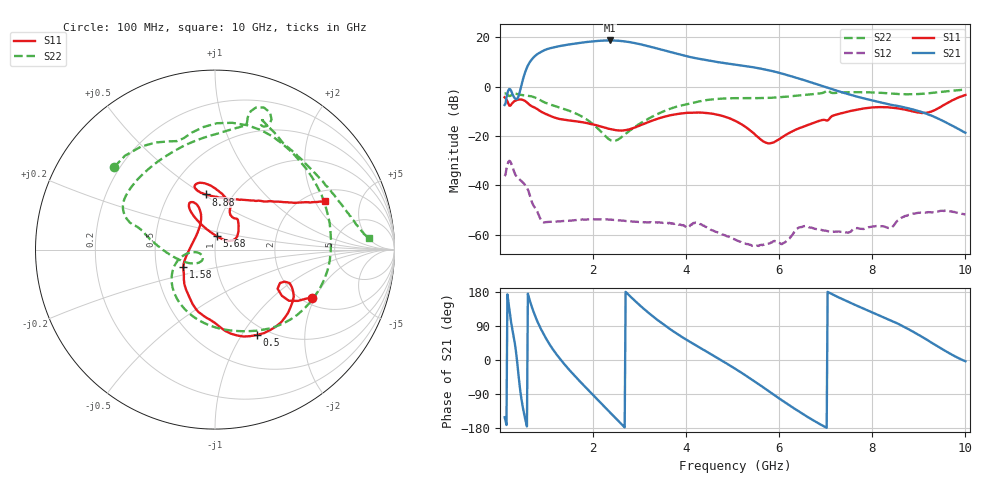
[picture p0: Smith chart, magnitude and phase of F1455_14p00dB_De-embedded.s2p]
! Integrated Device Technology
! Corporate Headquarters
! 6024 Silver Creek Valley Road
! San Jose, CA 95138  USA
! Phone:  1-408-284-8200
! Toll Free:  1-800-223-1366
! Webpage:  http://www.idt.com/
! Timing and RF Division
! 515 Groton Road, Suite 102
! Westford, MA 01886-6024
! Device:  F1455
! Description: 6-bit 0.5 dB Transmit Variable Gain Amplifier
! Frequency:  1400.0 -  2300.00 MHz
! Package:  6x6 mm Thin QFN Plastic Package: 28 pin
! State:  28
! Atten State:  14.0 dB
! Voltage:  +5.00 Volts
! Current:  217.654 mA
! Data:  The device was measured on a the F1455 evaluation board which has
!  individual transmission lines to the RF pins.  Data was collected
!  using a calibrated network analyzer.  The evaluation board was
!  de-embedded using a TRL calibration technique.
!  The reference plane is the edge of the package pin.
!  Pin  1 = CSb
!  Pin  2 = DATA
!  Pin  3 = CLK
!  Pin  4 = RSET
!  Pin  5 = GND
!  Pin  6 = RFIN  = Port 1
!  Pin  7 = GND
!  Pin  8 = NC
!  Pin  9 = NC
!  Pin 10 = NC
!  Pin 11 = NC
!  Pin 12 = NC
!  Pin 13 = NC
!  Pin 14 = /STBY
!  Pin 15 = GND
!  Pin 16 = RFOUT  = Port 2
!  Pin 17 = GND
!  Pin 18 = NC
!  Pin 19 = NC
!  Pin 20 = NC
!  Pin 21 = GND
!  Pin 22 = NC
!  Pin 23 = GND
!  Pin 24 = NC
!  Pin 25 = NC
!  Pin 26 = NC
!  Pin 27 = GND
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# GHz S dB R 50
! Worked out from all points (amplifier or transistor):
!   496 points, 100 MHz to 10 GHz, reference 50 ohm
!   highest |S21| = 18.7 dB at 2.36 GHz (marker M1)
!   |S21| within 3 dB of that: 1.109 GHz to 3.326 GHz (2.216 GHz wide, 99.9 % of centre)
!   unconditionally stable (mu >= 1): start of sweep to end of sweep
!   at 1.74 GHz: K = 29.23, MAG = 18.2 dB, |S12| = -54.0 dB
!   at 5.06 GHz: K = 147.19, MAG = 10.8 dB, |S12| = -62.2 dB
!   at 10 GHz: K = 236.73, MAG = -10.2 dB, |S12| = -51.9 dB
!   S11 on the Smith chart (normalised r, x): 100 MHz: 2.25, -1.90; 500 MHz: 0.89, -1.17; 1.58 GHz: 0.69, -0.14; 5.68 GHz: 1.01, +0.15; 8.88 GHz: 0.75, +0.51; 10 GHz: 2.46, +2.45
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0.1  -4.38 -26.4  -7.48 -151.1  -36.30 45.7  -2.78 140.8
0.38  -5.38 -40.8  -4.75 -17.4  -36.92 -114.9  -3.12 57.3
0.5  -5.51 -63.7  3.31 -130.7  -39.06 -153.0  -3.52 27.0
0.68  -7.96 -92.0  10.88 141.8  -46.50 144.3  -4.00 -15.3
0.8  -9.13 -107.4  13.10 103.0  -50.64 126.6  -4.84 -43.0
0.94  -10.74 -121.2  14.59 68.1  -55.06 123.7  -6.27 -69.4
1.24  -12.95 -140.4  16.21 11.0  -54.69 95.3  -8.28 -111.0
1.58  -13.96 -151.6  17.32 -38.4  -54.22 63.6  -10.52 -144.2
1.76  -14.45 -156.6  17.79 -61.9  -53.89 50.2  -12.15 -157.4
2.06  -15.63 -166.8  18.41 -99.8  -53.82 31.0  -16.26 -172.2
2.36  -17.22 174.8  18.67 -137.8  -53.96 14.3  -21.58 -162.6
2.56  -17.83 156.7  18.51 -162.9  -54.25 5.5  -21.23 -142.2
2.76  -17.46 137.3  18.08 172.6  -54.56 -2.3  -18.30 -142.2
3.06  -15.38 117.9  16.93 138.3  -54.96 -12.0  -14.45 -159.8
3.4  -13.00 111.1  15.29 104.3  -55.08 -22.5  -11.06 -178.3
4.08  -10.61 115.8  11.98 48.0  -56.56 -37.5  -6.94 163.6
5.06  -13.93 121.7  8.87 -23.5  -62.19 -80.0  -4.72 148.0
5.68  -22.49 82.3  6.96 -74.1  -64.14 -65.2  -4.66 122.9
6.7  -15.04 42.3  1.58 -156.9  -57.22 -131.3  -3.12 78.3
8.36  -8.46 106.9  -7.23 106.1  -57.33 156.8  -2.78 62.1
8.88  -10.14 99.2  -9.34 74.3  -51.51 142.7  -3.14 41.6
10  -3.44 23.9  -18.73 -3.4  -51.87 65.7  -1.28 4.4
